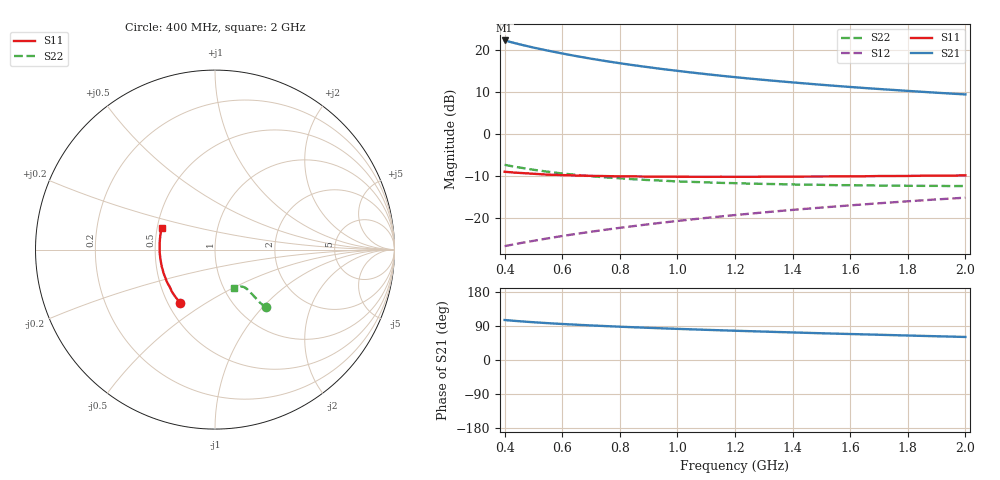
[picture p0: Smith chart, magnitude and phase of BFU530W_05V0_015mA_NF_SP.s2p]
! Filename:  P:\Prog\Test\Noise\ATS_data\Testdata_Net\06 Compressed Noise after Statistics\BFU530W_APM2013_09_A05_05p0V_015mA_NF_CM01_D.sf
! Date/Time: Tue 26/Mar/2013 18:06:05
! BFU530W_APM2013_09_A05_05p0V_1to25mA_NF_CM01_Bias7_R.sf
! Noise Parameter Data File
! BFU530W_APM2013_09_A05_05p0V_1to25mA_NF_CM01
! Date/time: Thu Mar 21 20:31:54 2013
! VAR V_out= 5.001000
! VAR I_out= 14.990000
! VAR V_in= 0.831900
! VAR I_in= 0.159100
! Device data file deembeded for feedlines and parallel
! Original file: \06 Compressed Noise after Statistics\BFU530W_APM2013_09_A05_05p0V_015mA_NF_CM01_R.sf
! Feed-files: PR019V01_070313_Feed1.s2p, PR019V01_070313_Feed2.s2p
! Parallel-file: PR019V01_070313_Par.s2p
# MHz S MA R 50
!  Freq-MHz  S11-mag  S11-arg  S21-mag  S21-arg  S12-mag  S12-arg  S22-mag  S22-arg
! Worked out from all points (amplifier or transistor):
!   37 points, 400 MHz to 2 GHz, reference 50 ohm
!   highest |S21| = 22.3 dB at 400 MHz (marker M1)
!   |S21| within 3 dB of that: start of sweep to 592.4 MHz
!   unconditionally stable (mu >= 1): 1.146 GHz to end of sweep
!   at 500 MHz: K = 0.83, MSG = 23.0 dB, |S12| = -25.5 dB
!   at 1.1 GHz: K = 1.00, MSG = 17.1 dB, |S12| = -20.0 dB
!   at 2 GHz: K = 1.01, MAG = 11.6 dB, |S12| = -15.2 dB
!   lowest NFmin = 0.87 dB at 420 MHz
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400  0.3539 -123.4  13.01 105.5  0.04593 62.9  0.4285 -48.8
420  0.3496 -126.2  12.48 104.2  0.04738 63.1  0.4157 -49.2
440  0.3453 -128.8  11.99 103.0  0.04884 63.3  0.4038 -49.4
480  0.3386 -133.5  11.11 100.7  0.05173 63.9  0.3837 -49.7
500  0.3352 -135.9  10.71 99.7  0.05315 64.1  0.374 -49.8
550  0.3266 -140.6  9.842 97.2  0.05691 64.8  0.3546 -49.9
600  0.3236 -145.1  9.101 95.0  0.0607 65.3  0.3377 -50.1
650  0.3194 -149.2  8.455 93.1  0.06444 65.8  0.3248 -50.2
700  0.3164 -152.9  7.891 91.2  0.06827 66.3  0.3134 -50.4
750  0.3144 -156.2  7.399 89.5  0.07208 66.7  0.3033 -50.4
800  0.3121 -159.4  6.966 87.9  0.07599 67.0  0.2961 -50.7
850  0.3115 -162.3  6.58 86.3  0.07984 67.3  0.2881 -50.9
950  0.3091 -167.3  5.928 83.5  0.08779 67.8  0.2771 -51.3
1050  0.3086 -171.9  5.393 80.9  0.09576 68.0  0.2683 -51.9
1150  0.3086 -176.2  4.946 78.4  0.1038 68.1  0.2609 -52.7
1200  0.3081 -178.1  4.755 77.2  0.1079 68.1  0.259 -53.3
1250  0.3082 180.0  4.572 76.1  0.1119 68.1  0.2557 -53.7
1350  0.3092 176.7  4.257 73.8  0.1202 68.0  0.2522 -54.8
1500  0.3108 171.7  3.855 70.6  0.1325 67.7  0.2474 -56.8
1650  0.313 167.3  3.527 67.6  0.1448 67.2  0.2436 -58.7
1750  0.3151 164.7  3.345 65.6  0.1532 66.8  0.2422 -60.2
2000  0.3209 158.2  2.958 60.8  0.174 65.6  0.2396 -64.5
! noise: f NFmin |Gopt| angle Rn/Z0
400  0.8875  0.1909  -178  0.0741
460  0.8982  0.2059  -177.5  0.0705
600  0.9128  0.1907  -175.2  0.0775
800  0.9504  0.2209  -171.3  0.0717
1000  0.9679  0.2311  -167  0.0731
1200  0.9919  0.2426  -163.9  0.0744
1400  1.013  0.2684  -162.2  0.0722
1600  1.021  0.3106  -157.3  0.0644
1800  1.073  0.2916  -155.1  0.0754
2000  1.082  0.3199  -155.9  0.0726
